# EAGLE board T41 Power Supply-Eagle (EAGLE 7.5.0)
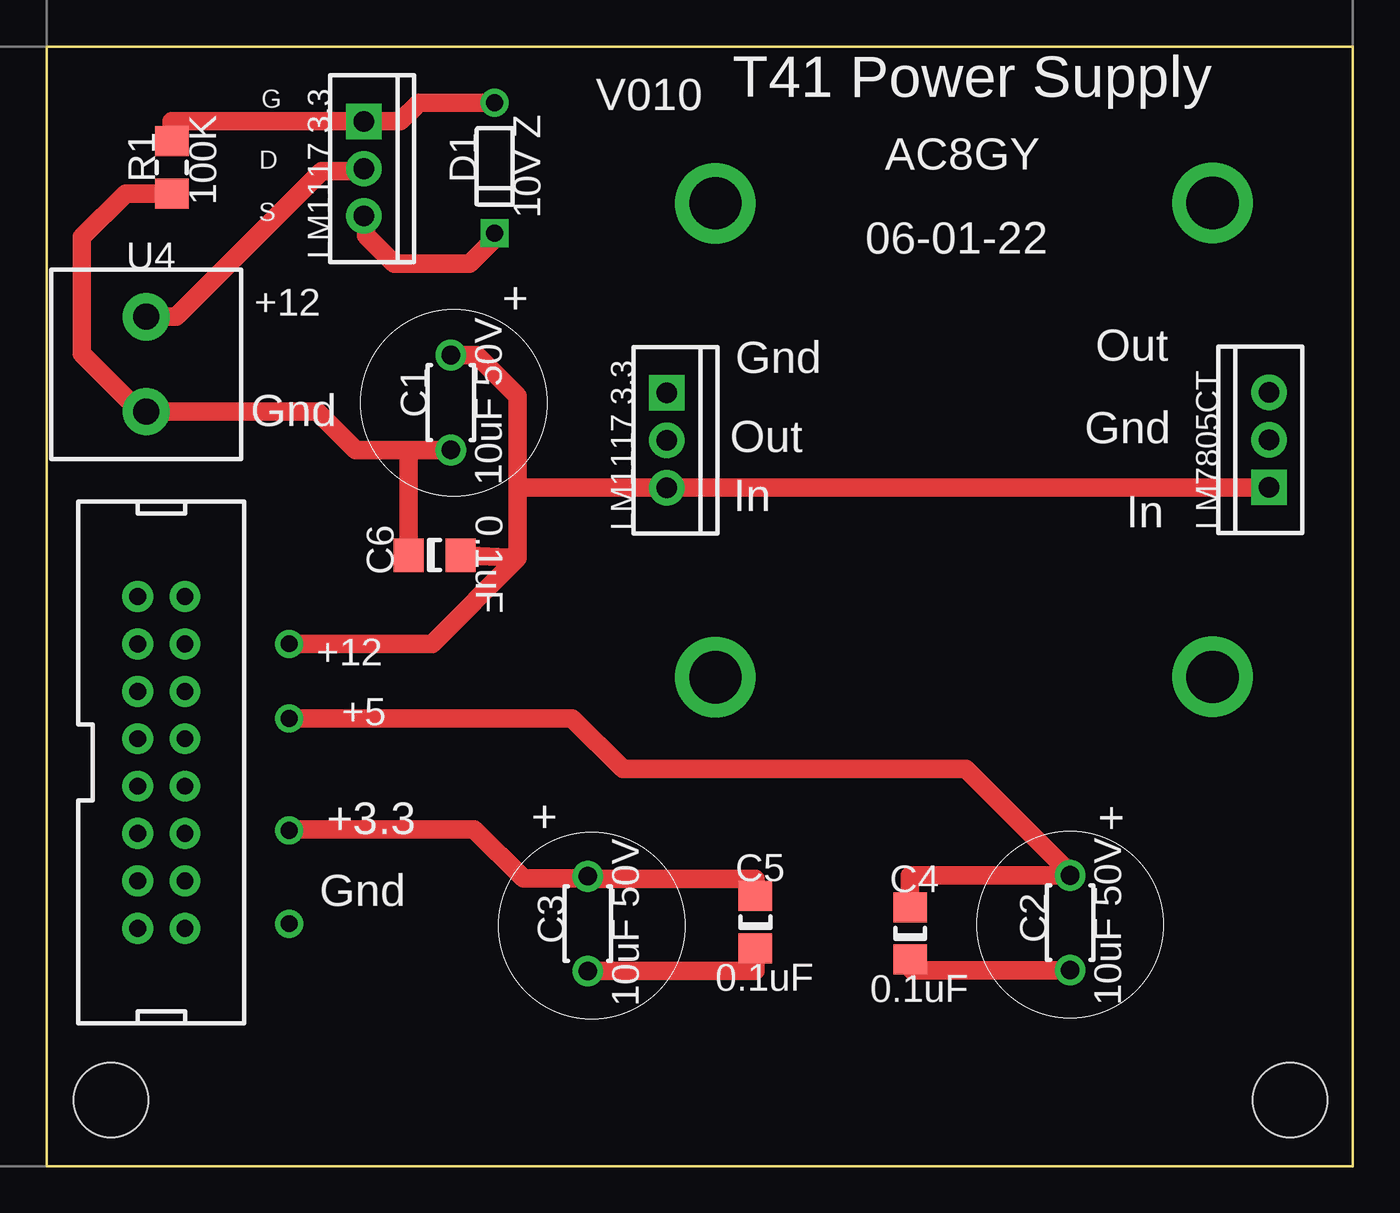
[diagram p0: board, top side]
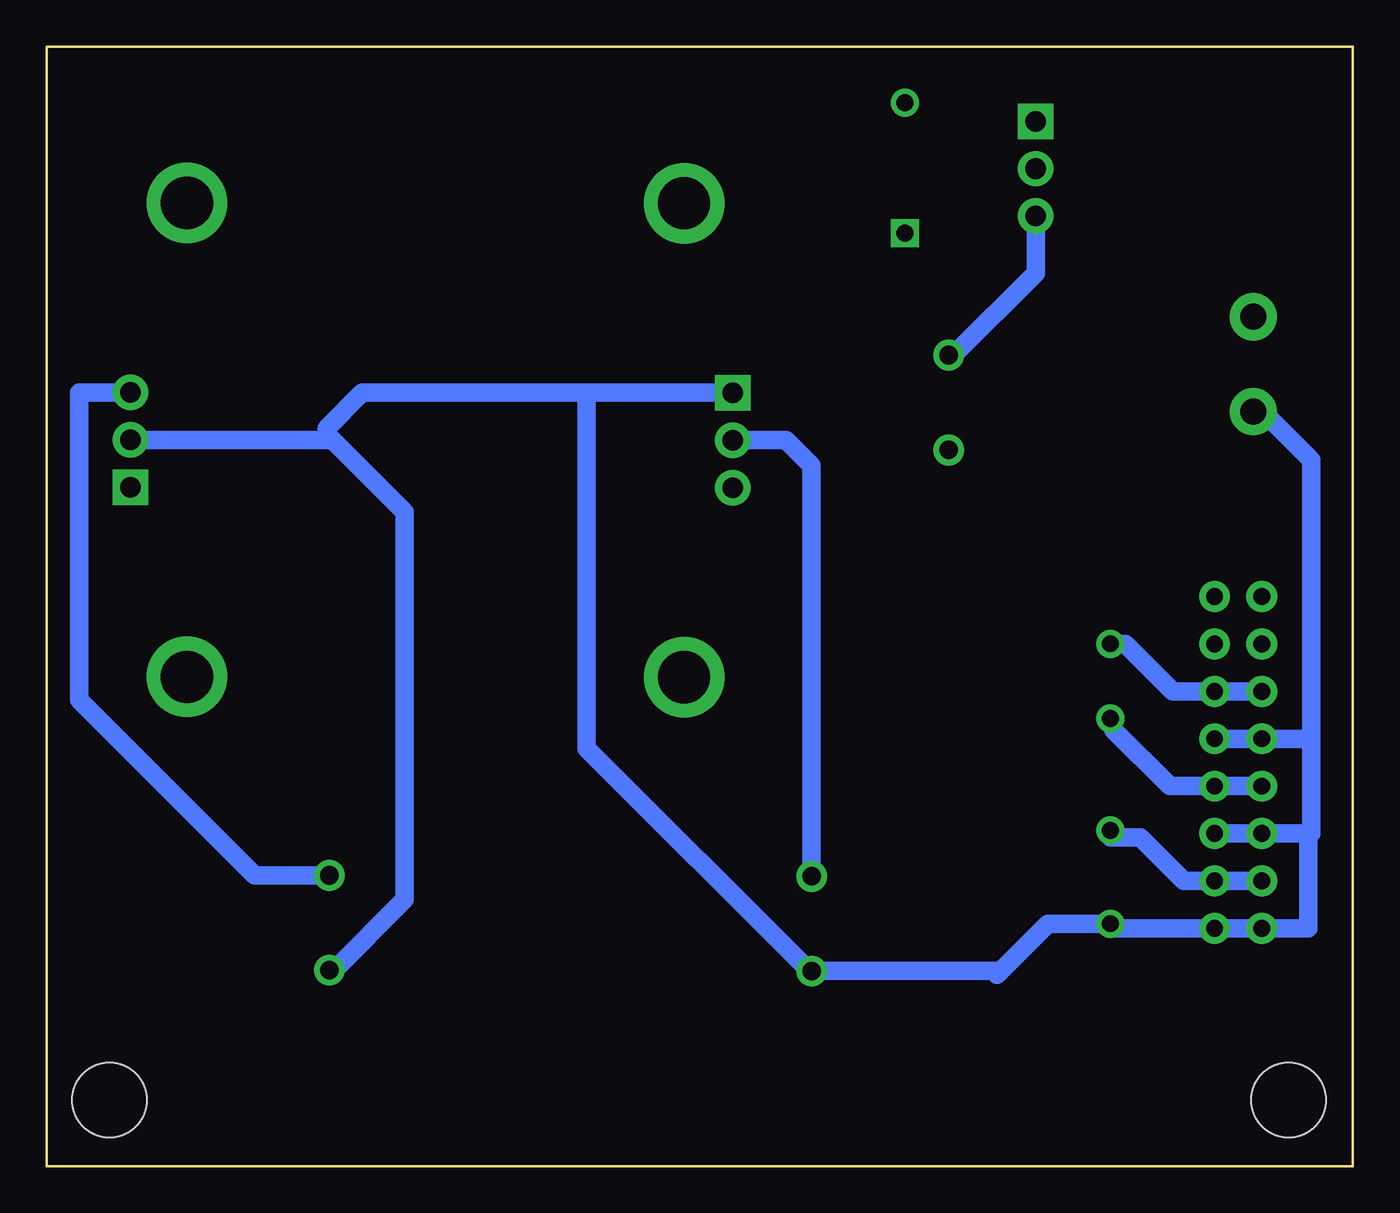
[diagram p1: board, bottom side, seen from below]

Size 70 x 60 mm. Coordinates in mm from the lower left corner, seen from the top.
Outline: 0,60 70,60 70,0 0,0 0,60
Copper layers (1*16): Top 0.035mm / dielectric 1.5mm / Bottom 0.035mm
Design rules "default *": minimum track width 10mil, minimum drill 0.61mm, track to track 8mil, track to pad 8mil, pad to pad 8mil, via to via 8mil, smd to smd 8mil, copper to edge 40mil, drill to drill 8mil, minimum pad ring 0mil, minimum via ring 8mil, stop-mask expansion 4mil, vias tented up to drill 19mil, thermal gap 10mil
Net classes: 0 Default: width 1 mm, clearance 0.5 mm, clearance 0.5 mm to class 1, clearance 0.5 mm to class 2; 1 Gnd: width 1.5 mm, clearance 0.5 mm, clearance 0.5 mm to class 0, clearance 0.5 mm to class 2; 2 Power: width 1.5 mm, clearance 0.5 mm, clearance 0.5 mm to class 0, clearance 0.5 mm to class 1
Holes 4 mm at 66.62,3.53 3.46,3.53

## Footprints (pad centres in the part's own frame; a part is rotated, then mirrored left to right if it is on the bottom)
P0 = drill 1 pad 1.65: 1 -2.54,0; 2 2.54,0
CAP_1206 = smd 1.6 x 1.8: 1 -1.4,0; 2 1.4,0
P6 = drill 0.9 pad 1.5 square: 1 0,0 | drill 0.9 pad 1.5: 2 7,0
Pad = drill 2.794 pad 4.318: 1 0,0
Pad_Pad9 = drill 0.9 pad 1.5: 1 0,0
IDC20M = drill 0.9 pad 1.651: 3 0,0
RES_1206 = smd 1.6 x 1.8: 1 -1.4,0; 2 1.4,0
TO-220 = drill 1.1 pad 1.9 square: 1 -2.54,0 | drill 1.1 pad 1.9: 2 0,0; 3 2.54,0
TO-220_U2 = drill 1.1 pad 1.9 square: 1 -2.54,0 | drill 1.1 pad 1.9: 2 0,0; 3 2.54,0
Power_conn = drill 1.397 pad 2.54: 1 -2.54,0; 2 2.54,0

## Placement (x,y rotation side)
C1  10uF 50V  [P0]  21.66,40.93 90 top
C2  10uF 50V  [P0]  54.85,13.05 90 top
C3  10uF 50V  [P0]  29,13 90 top
C4  0.1uF  [CAP_1206]  46.28,12.48 90 top
C5  0.1uF  [CAP_1206]  37.98,13.08 90 top
C6  0.1uF  [CAP_1206]  20.79,32.75 0 top
D1  10V Z  [P6]  24,50 90 top
Pad1  PAD  [Pad]  62.48,51.62 0 top
Pad2  PAD  [Pad]  62.48,26.22 0 top
Pad3  LM1117 3.3  [Pad]  35.84,51.61 0 top
Pad4  LM1117 3.3  [Pad]  35.84,26.21 0 top
Pad9  PAD  [Pad_Pad9]  13,13 0 top
Pad10  PAD  [Pad_Pad9]  13,18 0 top
Pad11  PAD  [Pad_Pad9]  13,24 0 top
Pad12  PAD  [Pad_Pad9]  13,28 0 top
PAD92  DEV_PAD92  [IDC20M]  4.87,27.99 90 top
PAD93  DEV_PAD93  [IDC20M]  4.87,25.45 90 top
PAD94  DEV_PAD94  [IDC20M]  4.87,22.91 90 top
PAD95  DEV_PAD95  [IDC20M]  4.87,20.37 90 top
PAD96  DEV_PAD96  [IDC20M]  4.87,17.83 90 top
PAD97  DEV_PAD97  [IDC20M]  4.87,15.29 90 top
PAD98  DEV_PAD98  [IDC20M]  4.87,12.75 90 top
PAD99  DEV_PAD99  [IDC20M]  7.41,12.75 90 top
PAD100  DEV_PAD100  [IDC20M]  7.41,15.29 90 top
PAD101  DEV_PAD101  [IDC20M]  7.41,17.83 90 top
PAD102  DEV_PAD102  [IDC20M]  7.41,20.37 90 top
PAD103  DEV_PAD103  [IDC20M]  7.41,22.91 90 top
PAD104  DEV_PAD104  [IDC20M]  7.41,25.45 90 top
PAD105  DEV_PAD105  [IDC20M]  7.41,27.99 90 top
PAD106  DEV_PAD106  [IDC20M]  7.41,30.53 90 top
PAD107  DEV_PAD107  [IDC20M]  4.87,30.53 90 top
R1  100K  [RES_1206]  6.71,53.53 90 top
U1  LM1117 3.3  [TO-220]  33.24,38.91 270 top
U2  LM7805CT  [TO-220_U2]  65.5,38.92 90 top
U3  MOSFET P Chan  [TO-220]  17,53.46 270 top
U4  POWER_CONN  [Power_conn]  5.33,42.98 90 top

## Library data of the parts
C1-C6 D1 Pad1-Pad4 Pad9-Pad12 PAD92-PAD107 R1 U3 U4 = common
U1 U2 = common; MANUFACTURER: National Semiconductor

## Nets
+3.3: C3.2 C5.2 Pad10.1 PAD97.13 PAD100.14 U1.2
+12: C1.1 C2.1 C3.1 C4.1 C5.1 C6.1 Pad9.1 PAD94.7 PAD96.11 PAD98.15 PAD99.16 PAD101.12 PAD103.8 R1.1 U1.1 U2.2 U4.1
Net_1: C2.2 C4.2 Pad11.1 PAD95.9 PAD102.10 U2.3
Net_4: C1.2 C6.2 D1.1 Pad12.1 PAD93.5 PAD104.6 U1.3 U2.1 U3.3
Net_5: U3.2 U4.2
Net_6: D1.2 R1.2 U3.1

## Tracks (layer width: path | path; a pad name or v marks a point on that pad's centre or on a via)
+3.3
  Top 1: Pad10.1 13,17.82 12.78,18.05 22.92,18.05 25.55,15.41 29.17,15.41 29.17,15.54 C3.2 29,15.39 37.98,15.39 C5.2
  Bottom 1: U1.2 30.37,38.91 29,37.54 C3.2 | 4.87,15.29 7.41,15.29 9.06,15.29 11.38,17.61 13,17.61 Pad10.1
+12
  Top 1: R1.1 4.23,52.13 1.89,49.79 1.89,43.55 4.99,40.44 U4.1 14.49,40.44 16.55,38.38 C1.1 19.39,38.38 C6.1 | C3.1 37.98,10.46 C5.1 | C4.1 46.36,11.08 46.36,10.51 C2.1
  Bottom 1: U1.1 41.06,41.45 | 41.06,41.45 41.06,22.4 29.12,10.46 C3.1 19.08,10.46 19.08,10.27 16.35,13 Pad9.1 13,12.75 7.41,12.75 4.87,12.75 2.4,12.75 2.4,17.83 | 7.41,17.83 4.87,17.83 2.4,17.83 | 2.23,22.91 4.87,22.91 7.41,22.91 | 2.23,22.91 2.23,17.83 2.4,17.83 | 41.06,41.45 53.09,41.45 55,39.54 55,39.25 | 55,39.25 55,38.92 U2.2 | 55,39.25 50.81,35.06 50.81,14.29 54.59,10.51 C2.1 | U4.1 4.83,40.44 2.23,37.84 2.23,22.91
Net_1
  Top 1: Pad11.1 28.17,24 30.88,21.29 49.27,21.29 54.85,15.7 C2.2 46.27,15.59 C4.2
  Bottom 1: 4.87,20.37 7.41,20.37 9.81,20.37 12.83,23.39 12.83,24 Pad11.1 | U2.3 68.25,41.46 68.25,25 58.85,15.59 C2.2
Net_4
  Top 1: C1.2 23.04,43.47 25.24,41.27 25.24,36.37 | 25.24,36.37 U1.3 65.5,36.37 U2.1 | Pad12.1 20.64,28 25.24,32.59 | 25.24,32.59 25.24,36.37 | C6.2 25.24,32.59 | U3.3 17.11,50.92 17.11,49.86 18.61,48.36 22.66,48.36 24,49.7 D1.1
  Bottom 1: 4.87,25.45 7.41,25.45 9.64,25.45 12.19,28 Pad12.1 | U3.3 17,47.87 21.41,43.47 C1.2
Net_5
  Top 1: U4.2 6.94,45.52 14.73,53.32 17,53.32 U3.2
Net_6
  Top 1: R1.2 6.71,56 U3.1 18.95,56 19.95,57 D1.2

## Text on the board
tPlace: T41 Power Supply | G | V010 | AC8GY | D | R1 | D1 | 100K | S | 10V Z | 06-01-22 | U4 | +12 | + | Out | Gnd | Gnd | C1 | Out | Gnd | In | 10uF 50V | In | 0.1uF | C6 | +12 | +5 | +3.3 | + | + | Gnd | C5 | C4 | C3 | C2 | 0.1uF | 0.1uF | 10uF 50V | 10uF 50V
